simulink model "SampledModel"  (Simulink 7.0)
settings: Solver=ode45  StartTime=0.0  StopTime=10.0  MaxStep=0.001  RelTol=1e-3
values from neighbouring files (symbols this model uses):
  T = 0.2    [AntennaAnalogico.m]    (also in Oscillations.m = 1; SampledDataSystem.m = 0.05)
  w1 = 5    [SampledDataSystem.m]
libraries: cstblocks x2

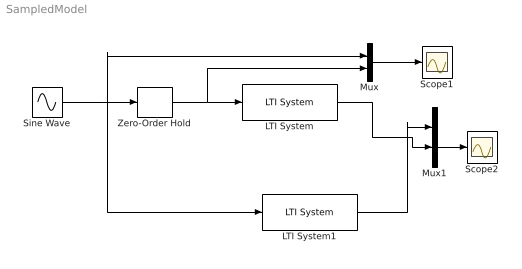
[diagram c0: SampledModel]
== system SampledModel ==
  LTI System : cstblocks/LTI System  SystemSampleTime=-1  sys=G  IC=[]
  LTI System1 : cstblocks/LTI System  SystemSampleTime=-1  sys=G  IC=[]
  Mux : Mux  Inputs=2
  Mux1 : Mux  Inputs=2
  Scope1 : Scope
  Scope2 : Scope
  Sine Wave : Sin  Frequency=w1  SampleTime=0
  Zero-Order Hold : ZeroOrderHold  SampleTime=T
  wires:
  Sine Wave/1 -> Zero-Order Hold/1, Mux/1, LTI System1/1
  Zero-Order Hold/1 -> LTI System/1, Mux/2
  Mux/1 -> Scope1/1
  Mux1/1 -> Scope2/1
  LTI System/1 -> Mux1/2
  LTI System1/1 -> Mux1/1
